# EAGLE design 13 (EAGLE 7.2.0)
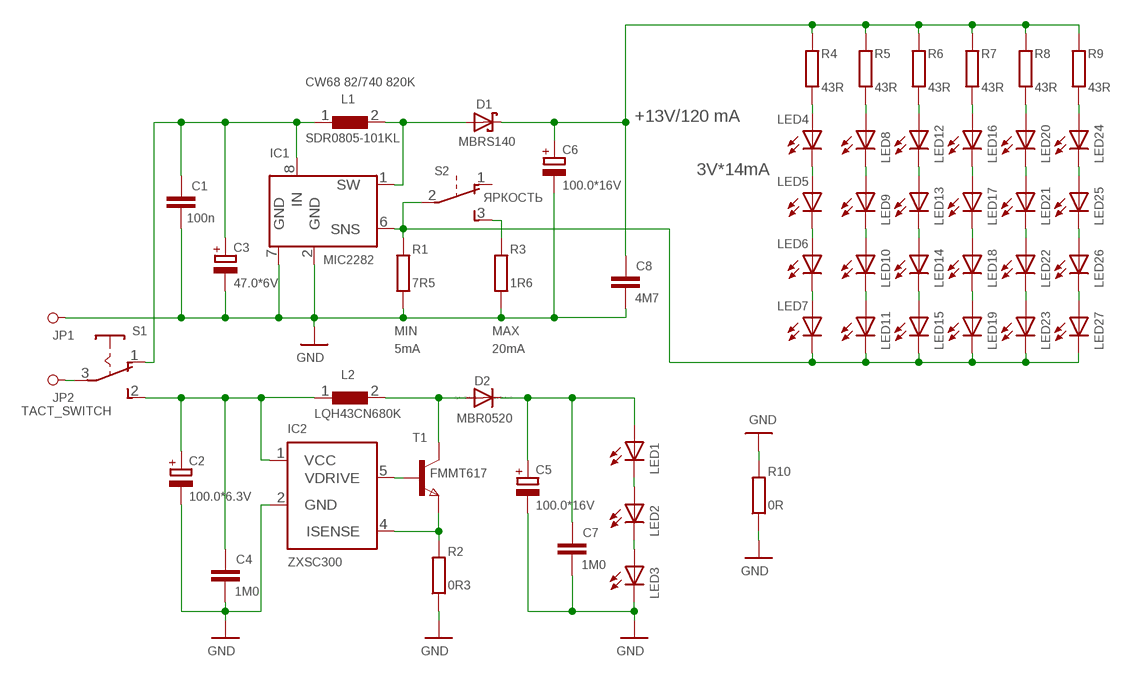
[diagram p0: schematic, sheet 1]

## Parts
C1  100n  C-EUC1206  [C1206]
C2  100.0*6.3V  CPOL-EUCT3528  [CT3528]
C3  47.0*6V  CPOL-EUB/3528-21W  [B/3528-21W]
C4  1M0  C-EUC1206  [C1206]
C5  100.0*16V  CPOL-EUCT3528  [CT3528]
C6  100.0*16V  CPOL-EUCT6032  [CT6032]
C7  1M0  C-EUC1206  [C1206]
C8  4M7  C-EUC1206  [C1206]
D1  MBRS140  MBRS130LT3  [SMB]
D2  MBR0520  MBR0520LT  [SOD123]
IC1  MIC2282  [MSOP-8]
IC2  ZXSC300  [SOT23-5]
JP1  PINHD-1X11.5X2.7_PISTONE  [1.5X2.7_PISTONE]
JP2  PINHD-1X11.5X2.7_PISTONE  [1.5X2.7_PISTONE]
L1  SDR0805-101KL  CHOKESDR0805  [SDR0805]
L2  LQH43CN680K  CHOKEC4532_1812  [C4532_1812]
LED1  LED5MM  [LED5MM]
LED2  LED5MM  [LED5MM]
LED3  LED5MM  [LED5MM]
LED4  LED5MM  [LED5MM]
LED5  LED5MM  [LED5MM]
LED6  LED5MM  [LED5MM]
LED7  LED5MM  [LED5MM]
LED8  LED5MM  [LED5MM]
LED9  LED5MM  [LED5MM]
LED10  LED5MM  [LED5MM]
LED11  LED5MM  [LED5MM]
LED12  LED5MM  [LED5MM]
LED13  LED5MM  [LED5MM]
LED14  LED5MM  [LED5MM]
LED15  LED5MM  [LED5MM]
LED16  LED5MM  [LED5MM]
LED17  LED5MM  [LED5MM]
LED18  LED5MM  [LED5MM]
LED19  LED5MM  [LED5MM]
LED20  LED5MM  [LED5MM]
LED21  LED5MM  [LED5MM]
LED22  LED5MM  [LED5MM]
LED23  LED5MM  [LED5MM]
LED24  LED5MM  [LED5MM]
LED25  LED5MM  [LED5MM]
LED26  LED5MM  [LED5MM]
LED27  LED5MM  [LED5MM]
R1  7R5  R-EU_R1206  [R1206]
R2  0R3  R-EU_R1206  [R1206]
R3  1R6  R-EU_R1206  [R1206]
R4  43R  R-EU_R1206  [R1206]
R5  43R  R-EU_R1206  [R1206]
R6  43R  R-EU_R1206  [R1206]
R7  43R  R-EU_R1206  [R1206]
R8  43R  R-EU_R1206  [R1206]
R9  43R  R-EU_R1206  [R1206]
R10  0R  R-EU_R1206  [R1206]
S1  TACT_SWITCH  [CHINA_NONAME]
S2  SS12F27  [SS12F27_HORIZ.]
T1  FMMT617  [SOT-23]

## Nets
GND: C1.2 C2.- C3.- C4.2 C5.- C6.- C7.2 C8.2 IC1.2(GND) IC1.7(GND) IC2.2(GND) JP1.1 LED3.K(C) R1.1 R2.1 R3.1 R10.1 R10.2
N$1: IC1.6(SNS) LED7.K(C) LED11.K(C) LED15.K(C) LED19.K(C) LED23.K(C) LED27.K(C) R1.2 S2.2(P)
N$2: C1.1 C3.+ IC1.8(IN) L1.1 S1.1(O)
N$3: D1.A IC1.1(SW) L1.2
N$4: C6.+ C8.1 D1.C R4.2 R5.2 R6.2 R7.2 R8.2 R9.2
N$6: R3.2 S2.3(S)
N$7: LED4.A R4.1
N$8: LED8.A R5.1
N$9: LED12.A R6.1
N$10: LED16.A R7.1
N$11: LED20.A R8.1
N$12: LED24.A R9.1
N$13: LED24.K(C) LED25.A
N$14: LED25.K(C) LED26.A
N$15: LED26.K(C) LED27.A
N$16: LED22.K(C) LED23.A
N$17: LED21.K(C) LED22.A
N$18: LED20.K(C) LED21.A
N$19: LED16.K(C) LED17.A
N$20: LED12.K(C) LED13.A
N$21: LED8.K(C) LED9.A
N$22: LED4.K(C) LED5.A
N$23: LED5.K(C) LED6.A
N$24: LED9.K(C) LED10.A
N$25: LED13.K(C) LED14.A
N$26: LED17.K(C) LED18.A
N$27: LED18.K(C) LED19.A
N$28: LED14.K(C) LED15.A
N$29: LED10.K(C) LED11.A
N$30: LED6.K(C) LED7.A
N$32: IC2.4(ISENSE) R2.2 T1.2(E)
N$33: LED2.K(C) LED3.A
N$34: LED1.K(C) LED2.A
N$35: IC2.5(VDRIVE) T1.3(B)
N$36: D2.A L2.2 T1.1(C)
N$37: C5.+ C7.1 D2.C LED1.A
N$38: C2.+ C4.1 IC2.1(VCC) L2.1 S1.2(S)
N$39: JP2.1 S1.3(P)
Unconnected: S2.1(O)

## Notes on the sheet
- CW68 82/740 820K
- +13V/120 mA
- 3V*14mA
- ЯРКОСТЬ
- MIN | MAX
- 5mA | 20mA

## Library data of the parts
C1 C4 C7 C8 = rcl:C-EU: CAPACITOR, European symbol
C2 C3 C5 C6 = rcl:CPOL-EU: POLARIZED CAPACITOR, European symbol
D1 = diode:MBRS130LT3: Schottky Power Rectifier
D2 = diode:MBR0520LT: SCHOTTKY BARRIER RECTIFIER
IC1 = my_ics:MIC2282
IC2 = zetex:ZXSC300: SINGLE OR MULTI CELL LED DRIVER SOLUTION Manufacturer: http://www.zetex.com http://www.avxcorp.com http://www.coilcraft.com http://www.nichia.co.jp Source: http://www.zetex.com/3.0/pdf/ZXSC300.pdf; MPN: ZXSC300E5TA; OC_FARNELL: 7721340; OC_NEWARK: 34M9011
JP1 JP2 = R2D2:PINHD-1X1: PIN HEADER
L1 L2 = my_inductors:CHOKE
LED1-LED27 = led:LED: LED
R1-R10 = rcl:R-EU_: RESISTOR, European symbol
S1 = my_switch:TACT_SWITCH
S2 = my_switch:SS12F27
T1 = zetex:FMMT6*: NPN SILICON POWER (SWITCHING) TRANSISTORS SuperSOT Source: http://www.zetex.com/3.0/pdf/FMMT617.pdf; MPN: FMMT617; OC_FARNELL: 9526420; OC_NEWARK: 96K9966

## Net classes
0 default: clearance 0.205 mm

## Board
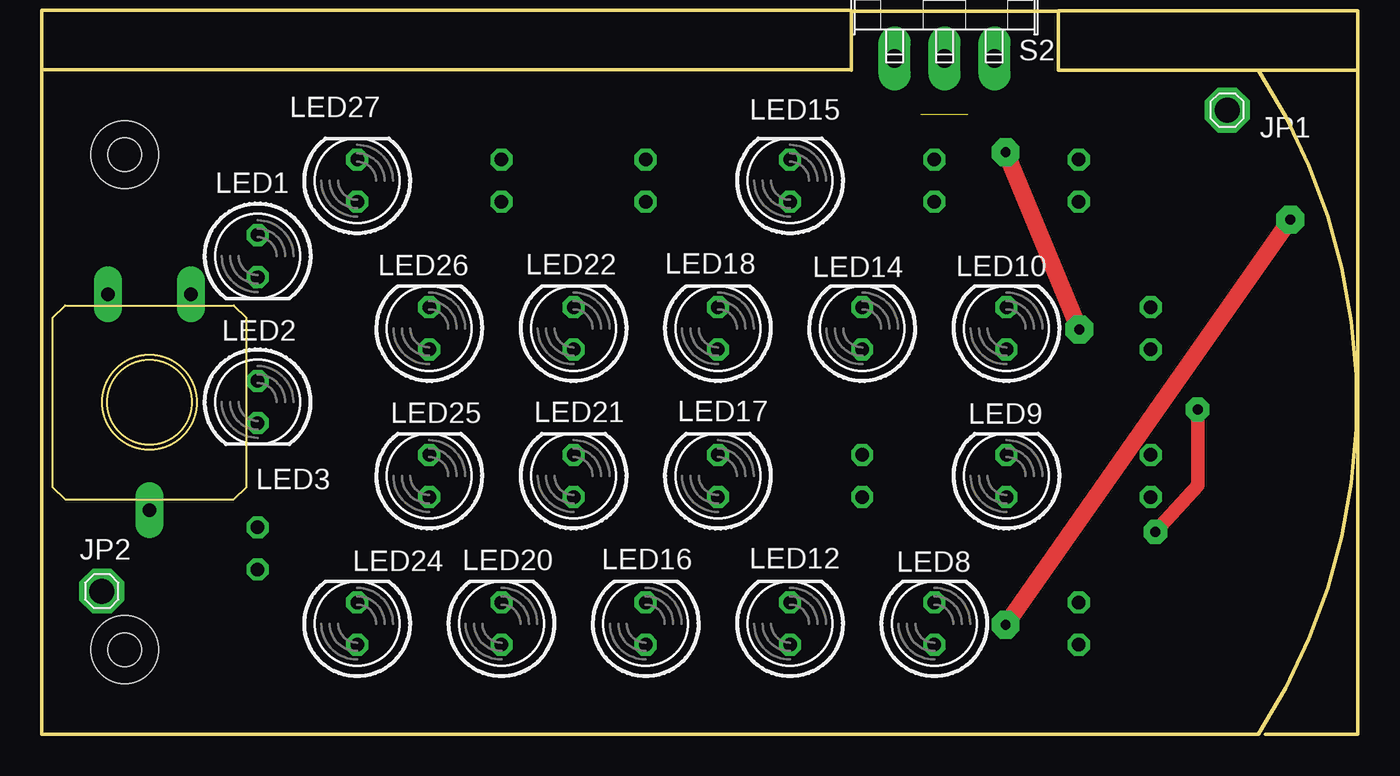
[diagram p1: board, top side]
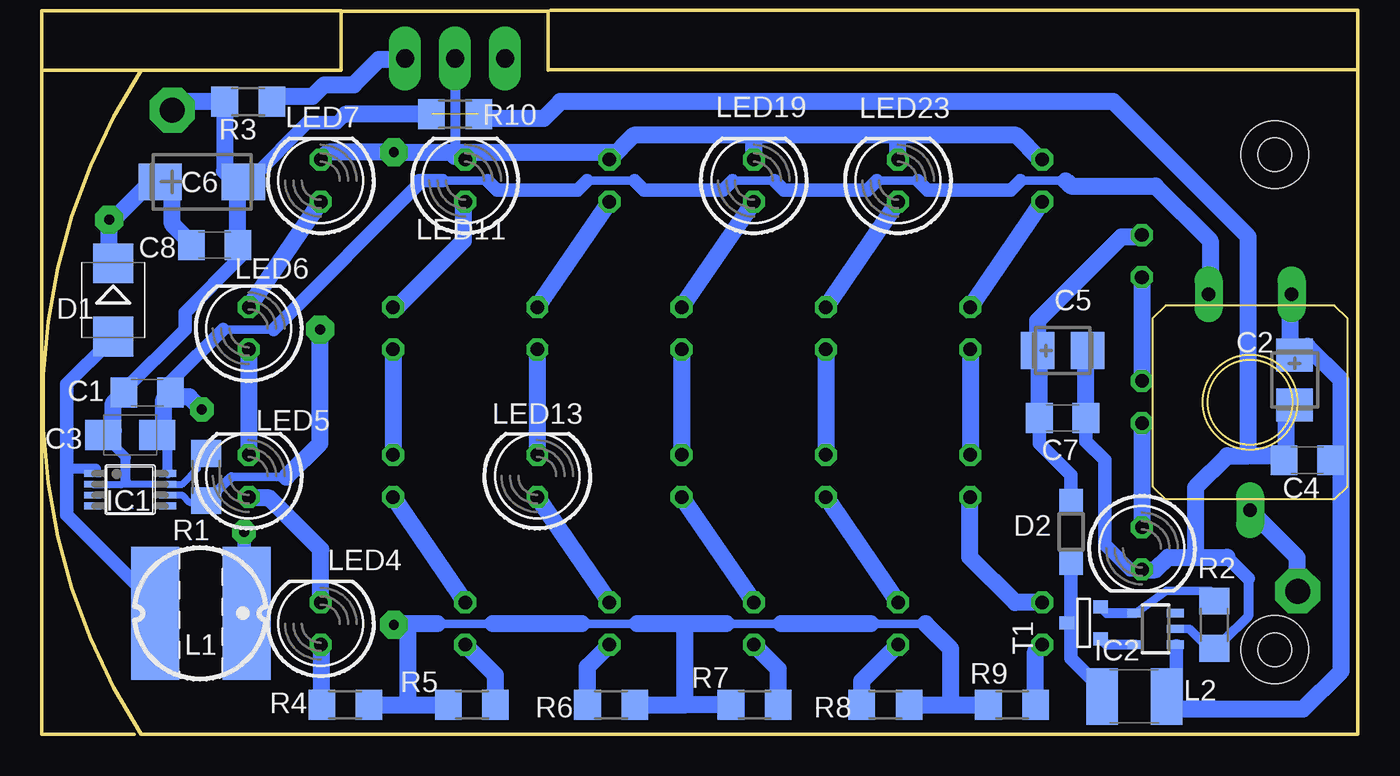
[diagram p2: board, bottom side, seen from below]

Size 78.6 x 25.83 mm. Coordinates in mm from the lower left corner, seen from the top.
Outline: 78.6,0 73.01,0
Copper layers (1*16): Top 0.035mm / dielectric 1.5mm / Bottom 0.035mm
Design rules "default": minimum track width 10mil, minimum drill 24mil, track to track 8mil, track to pad 8mil, pad to pad 8mil, via to via 8mil, smd to smd 8mil, copper to edge 40mil, drill to drill 8mil, minimum pad ring 10mil, minimum via ring 8mil, stop-mask expansion 4mil, vias tented up to drill 0mil, thermal gap 10mil
Holes 2 mm at 4.35,34.9 4.35,5.1
Holes 4.06 mm at 4.35,34.9 4.35,5.1
Milling: 13 lines

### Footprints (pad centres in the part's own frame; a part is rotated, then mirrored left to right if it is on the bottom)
C1206 = smd 1.6 x 1.8: 1 -1.4,0; 2 1.4,0
CT3528 = smd 2 x 2.2: + -1.5,0; - 1.5,0
B/3528-21W = smd 2.15 x 1.8: + 1.625,0; - -1.625,0
CT6032 = smd 2.6 x 2.2: + -2.5,0; - 2.5,0
SMB = smd 2.4 x 2.4: A 2.2,0; C -2.2,0
SOD123 = smd 1.4 x 1.4: A 1.9,0; C -1.9,0
MSOP-8 = smd 0.4 x 1.016: 1 -0.98,-2.263; 4 0.98,-2.263; 5 0.975,2.263; 8 -0.98,2.263 | smd 0.406 x 1.016: 2 -0.325,-2.263; 3 0.325,-2.263; 6 0.325,2.263; 7 -0.325,2.263
SOT23-5 = smd 0.5 x 1: 1 -0.95,-1.2; 2 0,-1.2; 3 0.95,-1.2; 4 0.95,1.2; 5 -0.95,1.2
1.5X2.7_PISTONE = drill 1.5 pad 2.7 octagon: 1 0,0
SDR0805 = smd 2.9 x 8: 1 -2.757,0; 2 2.748,0.001
C4532_1812 = smd 1.9 x 3.4: 1 -1.95,0; 2 1.95,0
LED5MM = drill 0.813 octagon: A -1.27,0; K 1.27,0
R1206 = smd 1.6 x 1.803: 1 -1.422,0; 2 1.422,0
CHINA_NONAME = drill 0.8 pad 1.676 long: 1 -6.5,2.5; 2 -6.5,-2.5; 3 6.5,0
SS12F27_HORIZ. = drill 1.1 pad 1.93 long: 1 -3.01,-4.255; 2 0,-4.255; 3 3.01,-4.255
SOT-23 = smd 0.787 x 0.889: 1 0.025,-1.016; 2 -0.94,1.016; 3 0.991,1.016

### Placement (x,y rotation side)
C1  72.25,20.57 180 bottom
C2  3.16,21.34 270 bottom
C3  73.26,18.03 0 bottom
C4  2.4,16.51 180 bottom
C5  17.13,23.11 0 bottom
C6  68.95,33.27 0 bottom  (outside the outline)
C7  17.13,19.05 0 bottom
C8  68.18,29.46 0 bottom  (outside the outline)
D1  74.28,26.16 270 bottom
D2  16.62,12.19 270 bottom
IC1  73.26,14.73 270 bottom
IC2  11.54,6.35 90 bottom
JP1  70.72,37.59 0 top  (outside the outline)
JP2  2.98,8.62 0 top
L1  69,7.29 180 bottom
L2  12.81,2.29 180 bottom
LED1  12.36,28.8 270 top
LED2  12.36,20.01 270 top
LED3  12.35,11.19 270 bottom
LED4  61.78,6.67 90 bottom
LED5  66.13,15.56 90 bottom
LED6  66.13,24.45 90 bottom
LED7  61.78,33.34 90 bottom  (outside the outline)
LED8  53.1,6.67 90 top
LED9  57.44,15.56 90 top
LED10  57.44,24.45 90 top
LED11  53.1,33.34 90 bottom  (outside the outline)
LED12  44.41,6.67 90 top
LED13  48.75,15.56 90 bottom
LED14  48.75,24.45 90 top
LED15  44.41,33.34 90 top  (outside the outline)
LED16  35.72,6.67 90 top
LED17  40.07,15.56 90 top
LED18  40.07,24.45 90 top
LED19  35.72,33.34 90 bottom  (outside the outline)
LED20  27.04,6.67 90 top
LED21  31.38,15.56 90 top
LED22  31.38,24.45 90 top
LED23  27.04,33.34 90 bottom  (outside the outline)
LED24  18.35,6.67 90 top
LED25  22.69,15.56 90 top
LED26  22.69,24.45 90 top
LED27  18.35,33.34 90 top  (outside the outline)
R1  68.69,15.49 270 bottom
R2  7.99,6.6 90 bottom
R3  66.15,38.1 0 bottom  (outside the outline)
R4  60.31,1.78 0 bottom
R5  52.69,1.78 180 bottom
R6  44.31,1.78 0 bottom
R7  35.67,1.78 180 bottom
R8  27.8,1.78 0 bottom
R9  20.18,1.78 180 bottom
R10  53.71,37.34 0 bottom  (outside the outline)
S1  5.84,19.99 270 top
S2  53.71,44.96 0 top  (outside the outline)
T1  15.86,6.73 270 bottom

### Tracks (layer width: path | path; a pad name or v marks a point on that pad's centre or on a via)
GND  (1 unrouted)
  Bottom 0.406: R1.1 69.2,16.15 69.2,16 70.15,15.06 IC1.7 73.59,15.06 73.52,15.24 73.7,15.06 IC1.2 | 67.17,33.53 66.66,33.49 | 12.33,9.91 12.35,9.91 LED3.K
  Bottom 0.508: R2.1 8.14,5.33 8.49,5.33 9.51,6.35 IC2.2
  Bottom 0.61: 73.52,15.24 73.52,16.66 C3.- | 12.05,9.91 12.33,9.91 | 5.95,9.4 5.95,7.11 7.48,5.59
  Bottom 0.813: C3.- 74.53,18.03 74.28,18.29 | C1.2 73.65,20.7 69.96,24.38 69.96,25.4 66.66,28.7 66.66,29.34 C8.2 | 66.78,32.94 C6.- | 7.48,5.59 7.58,5.59 R2.1 | C7.2 15.73,17.65 14.59,16.51 14.59,11.43 13.07,9.91 12.37,9.91 LED3.K | 7.22,10.67 5.95,9.4 | 9.13,10.79 9.26,10.67 | 60.31,37.34 60.82,36.83 62.6,36.83 65.9,33.53 | 65.9,33.53 66.19,33.53 C6.- | C6.- 66.15,33.27 65.9,33.53
  Bottom 1.016: 67.17,33.53 67.57,33.93 R3.1 70.22,38.1 JP1.1 | 66.66,33.49 C6.- | 74.28,18.29 74.28,19.94 C1.2 | C8.2 66.78,32.94 | 3.8,16.39 3.92,16.51 | 3.92,16.51 4.18,16.76 | 4.18,16.76 5.95,16.76 | 4.18,16.76 3.67,16.76 3.67,19.58 C2.- | 12.33,9.91 11.54,9.91 10.78,10.67 9.26,10.67 7.22,10.67 | 9.13,10.79 9.13,14.86 7.22,16.76 5.95,16.76 | C7.2 15.73,23.01 C5.- | C4.2 3.92,16.51 | 5.95,16.76 5.95,29.97 14.08,38.1 47.36,38.1 48.37,37.08 52.03,37.08 R10.2 | R10.1 60.31,37.34
N$1  (via drill 0.6 pad 1.68)
  Top 1.016: v61.83,24.38 v57.39,35.05
  Bottom 0.406: IC1.6 70.15,14.41 69.71,13.97 68.84,13.97 R1.2
  Bottom 0.508: 68.84,13.97 68.69,13.97 | 67.17,15.49 63.87,15.49
  Bottom 0.61: 68.69,13.97 67.17,15.49 | S2.2 53.71,34.8
  Bottom 1.016: LED27.K 18.46,34.61 19.92,36.07 27.04,36.07 | 27.04,36.07 35.67,36.07 | 35.67,36.07 42.95,36.07 LED15.K 44.09,35.05 52.94,35.05 | LED7.K 61.58,34.81 61.33,35.05 v57.39,35.05 52.94,35.05 | LED19.K 35.72,36.02 35.67,36.07 | LED23.K 27.04,36.07 | 63.87,15.49 61.83,17.53 v61.83,24.38 | 52.94,35.05 52.94,34.76 LED11.K 53.2,34.71 53.71,34.8 52.94,35.05
N$2  (via drill 0.6 pad 1.42)
  Top 0.813: v66.41,12.19 68.95,14.99 v68.95,19.56
  Bottom 0.406: 17.07,33.34 16.94,33.34 | 71,17.4 C3.+ 71.49,18.03 | 70.72,20.2 C1.1
  Bottom 0.508: 54.47,33.34 51.74,33.34 | 45.77,33.34 42.91,33.34 | 37.01,33.34 34.47,33.34 | 28.31,33.34 25.83,33.34 | 19.67,33.34 17.07,33.34 | 67.68,24.38 64.63,24.38
  Bottom 0.61: 8.24,27.41 S1.1 | IC1.8 71,17.4
  Bottom 0.813: 51.74,33.34 51.17,32.77 46.34,32.77 45.77,33.34 | 42.91,33.34 42.34,32.77 37.58,32.77 37.01,33.34 | 34.47,33.34 33.89,32.77 28.88,32.77 28.31,33.34 | 25.83,33.34 25.26,32.77 20.24,32.77 19.67,33.34 | 8.34,27.53 S1.1 | 70.72,20.2 70.72,21.34 67.68,24.38 | 64.63,24.38 55.74,33.27 | 55.74,33.27 55.68,33.34 | L1.1 66.25,8.73 66.41,8.89 v66.41,12.19 | 70.09,20.32 C1.1 71.23,20.19 | 71.49,18.03 71.49,18.29 71.23,18.54 | 55.74,33.27 55.93,33.27 55.87,33.34 55.68,33.34 | 55.68,33.34 54.47,33.34
  Bottom 1.016: 16.94,33.34 16.62,33.02 11.54,33.02 8.24,29.72 8.24,27.41 | v68.95,19.56 69.71,20.32 70.09,20.32 | 71.23,18.54 71.23,20.19
N$3
  Bottom 0.406: 75.31,16 IC1.1 | 74.53,23.62 73.86,23.62 D1.A
  Bottom 0.61: 77.07,16 75.31,16 | 71.99,8.13 71.99,7.53 L1.2
  Bottom 0.813: 74.53,23.62 77.07,21.08 77.07,16 77.07,13.21 71.99,8.13
N$4  (via drill 0.6 pad 1.68)
  Top 1.016: v57.39,6.6 v74.53,30.99
  Bottom 0.508: 25.39,6.67 28.69,6.67 | 34.08,6.67 37.39,6.67 | 42.72,6.67 46.09,6.67 | 51.42,6.67 54.79,6.67
  Bottom 1.016: R4.2 56.56,1.78 | 56.56,1.78 R5.2 | R6.2 39.86,1.78 | 23.86,1.78 R9.2 | R8.2 23.86,1.78 | 23.86,1.78 23.86,5.14 25.39,6.67 | R7.2 39.86,1.78 | 39.86,1.78 39.86,6.67 | 28.69,6.67 34.08,6.67 | 39.86,6.67 42.72,6.67 | 46.09,6.67 51.42,6.67 | 37.39,6.67 39.86,6.67 | 56.56,6.67 56.56,1.78 | 54.79,6.67 56.56,6.67 | 56.56,6.67 56.75,6.67 v57.39,6.6 | C8.1 69.58,29.59 70.72,30.73 70.72,33.02 71.19,33.02 C6.+ 71.99,33.27 74.28,30.99 v74.53,30.99 74.53,28.45 74.45,28.36 D1.C
N$6
  Bottom 1.016: R3.2 64.41,38.42 62.28,38.42 61.58,39.12 59.8,39.12 58.28,40.64 56.78,40.64 S2.3
N$7
  Bottom 1.016: R4.1 61.73,5.35 LED4.A
N$8
  Bottom 1.016: R5.1 51.27,3.57 LED8.A
N$9
  Bottom 1.016: R6.1 45.73,4.08 LED12.A
N$10
  Bottom 1.016: R7.1 34.25,3.92 LED16.A
N$11
  Bottom 1.016: R8.1 29.22,3.21 LED20.A
N$12
  Bottom 1.016: R9.1 18.76,4.99 LED24.A
N$13
  Bottom 1.016: LED24.K 19.99,7.94 22.72,10.67 22.72,14.26 LED25.A
N$14
  Bottom 1.016: LED26.A LED25.K
N$15
  Bottom 1.016: LED26.K LED27.A
N$16
  Bottom 1.016: LED23.A LED22.K
N$17
  Bottom 1.016: LED22.A LED21.K
N$18
  Bottom 1.016: LED21.A LED20.K
N$19
  Bottom 1.016: LED17.A LED16.K
N$20
  Bottom 1.016: LED13.A LED12.K
N$21
  Bottom 1.016: LED9.A LED8.K
N$22
  Bottom 1.016: LED4.K 61.78,11.12 64.88,14.22 66.06,14.22 LED5.A
N$23
  Bottom 1.016: LED6.A LED5.K
N$24
  Bottom 1.016: LED10.A LED9.K
N$25
  Bottom 1.016: LED14.A LED13.K
N$26
  Bottom 1.016: LED18.A LED17.K
N$27
  Bottom 1.016: LED19.A LED18.K
N$28
  Bottom 1.016: LED15.A LED14.K
N$29
  Bottom 1.016: LED10.K 57.2,25.72 53.2,29.72 53.2,31.97 LED11.A
N$30
  Bottom 1.016: LED7.A LED6.K
N$32
  Bottom 0.508: R2.2 7.99,8.38 8.24,8.64 10.9,8.64 IC2.4
  Bottom 0.61: IC2.4 14.47,7.3 T1.2
N$33
  Bottom 1.016: LED2.K 12.36,12.47 LED3.A
N$34
  Bottom 1.016: LED1.K LED2.A
N$35
  Bottom 0.61: IC2.5 14.5,5.4 T1.3
N$36
  Bottom 0.813: L2.2 14.84,2.37 14.84,2.79 16.62,4.57 16.62,6.48 16.85,6.71 T1.1 16.62,6.73 | 16.62,6.6 16.62,6.73 | 16.62,6.73 D2.A
N$37
  Bottom 0.406: 18.4,18.92 C7.1 | 18.53,23.01 C5.+
  Bottom 0.813: D2.C 16.62,15.62 18.53,17.53 C7.1 | 12.46,29.97 LED1.A
  Bottom 1.016: C7.1 18.53,23.01 | C5.+ 18.63,24.92 13.57,29.97 12.46,29.97
N$38
  Bottom 0.508: IC2.1 10.27,5.33
  Bottom 0.813: 10.27,5.33 10.27,1.52
  Bottom 1.016: L2.1 10.86,1.61 10.78,1.52 10.27,1.52 2.65,1.52 0.37,3.81 0.37,16.26 | C4.1 0.37,16.26 | 0.37,16.26 0.37,21.34 2.4,23.37 3.16,23.11 | 3.16,23.11 3.41,23.37 3.41,26.42 S1.2 | 3.16,23.11 C2.+
N$39
  Bottom 1.016: JP2.1 3,10.65 S1.3
(copper drawn outside any net)
  shapes: Bottom area x1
